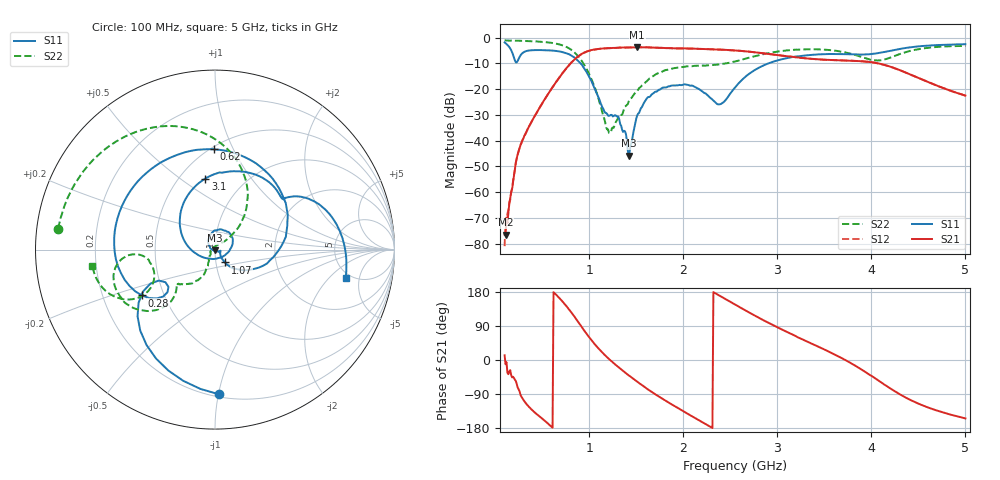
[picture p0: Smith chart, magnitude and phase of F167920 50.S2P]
!  2-Port S-parameters saved by WinCal
! VAR MeasName=S-Parameters (CALIBRATED_DATA) read from VNA (N5242A)
! VAR MeasDate=2016-11-22 9:57:59
! VAR NAME=F167920 50
! VAR FILENAME=F167920 50.S2P
! VAR DATE=2016-11-22 9:57:59
! VAR PHYS_PORTS=1,2
# Hz S DB R 50
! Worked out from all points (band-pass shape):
!   491 points, 100 MHz to 5 GHz, reference 50 ohm
!   highest |S21| = -3.74 dB at 1.51 GHz (marker M1); lowest = -76.6 dB at 110 MHz (marker M2)
!   |S21| within 3 dB of the highest: 903.5 MHz to 2.992 GHz (2.088 GHz wide, 107 % of centre)
!   lowest |S11| = -45.8 dB at 1.42 GHz (marker M3), VSWR 1.01, Z = 50.1 - j0.498 ohm
!   |S11| at or under -10 dB: 906.9 MHz to 2.905 GHz (1.998 GHz wide, 105 % of centre)
!   |S22| runs from -37.0 to -1.1 dB; largest |S21 - S12| = 0.0019
!   S11 on the Smith chart (normalised r, x): 100 MHz: 0.22, -1.01; 280 MHz: 0.38, -0.25; 620 MHz: 0.52, +0.84; 1.07 GHz: 1.10, -0.16; 3.1 GHz: 0.66, +0.63; 5 GHz: 4.50, -3.19
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1e8  -1.86 -88.2  -76.49 12.4  -80.99 9.0  -1.10 172.4
1.1e8  -2.15 -96.0  -76.55 -11.4  -71.80 -81.2  -1.10 171.6
2e8  -7.83 -152.2  -53.36 -47.5  -53.09 -46.1  -1.17 164.7
2.8e8  -6.36 -147.9  -40.73 -97.2  -40.84 -97.0  -1.24 158.3
4.1e8  -4.86 158.7  -31.11 -136.0  -31.10 -135.8  -1.43 146.6
6.2e8  -5.06 90.7  -18.68 179.0  -18.69 179.0  -2.15 121.4
7.9e8  -6.53 33.2  -10.48 132.1  -10.48 132.2  -4.27 89.5
9.2e8  -10.46 -15.0  -6.31 87.3  -6.31 87.4  -9.06 58.8
1.07e9  -20.87 -52.4  -4.54 38.3  -4.54 38.3  -20.43 40.4
1.21e9  -30.37 -19.4  -4.09 2.6  -4.09 2.6  -37.01 119.4
1.3e9  -30.72 -18.9  -3.95 -16.7  -3.95 -16.7  -31.73 -160.4
1.42e9  -45.82 -76.4  -3.85 -40.7  -3.85 -40.7  -24.76 -120.7
1.51e9  -30.20 156.9  -3.74 -57.3  -3.74 -57.3  -20.74 -114.7
1.74e9  -20.25 99.0  -3.95 -96.3  -3.96 -96.3  -13.73 -121.5
2.09e9  -18.60 34.8  -4.24 -148.1  -4.25 -148.1  -11.12 -136.8
2.38e9  -25.91 -75.2  -4.61 170.6  -4.62 170.6  -10.40 -135.1
2.55e9  -19.38 -167.6  -4.97 146.5  -4.97 146.6  -9.28 -131.1
3.1e9  -7.97 97.7  -7.21 74.3  -7.24 74.3  -4.97 -145.4
3.37e9  -6.68 69.1  -8.26 42.6  -8.28 42.8  -4.52 -159.2
3.85e9  -6.57 38.6  -9.05 -18.1  -9.06 -17.9  -6.98 -176.7
4.19e9  -5.20 32.6  -11.15 -73.3  -11.17 -73.0  -7.91 -150.5
5e9  -2.56 -12.3  -22.51 -154.1  -22.52 -153.9  -3.24 -172.6
